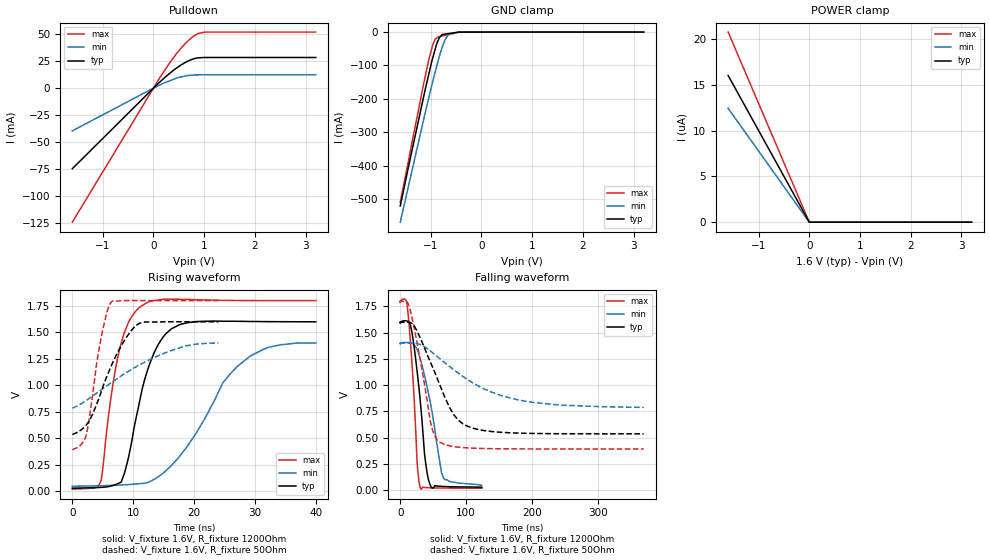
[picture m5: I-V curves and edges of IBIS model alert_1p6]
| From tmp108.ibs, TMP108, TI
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|   alert_1p6 Model
[Model]   alert_1p6
Model_type   Open_drain
Polarity   Non-Inverting
Vmeas = 0.8
Vref = 1.6
Cref = 2pF
Rref = 1200
|   typ   min   max
C_comp   9.597e-13   9.560e-13   1.010e-12
| Where nom  PVT is Nominal Process, 1.6V, 27C
|   Fast PVT is Strong Process,  1.8V, -40C
|   Slow PVT is Weak Process,   1.4V, 125C
[Voltage Range]   1.6   1.4   1.8
|Ambient Temperature   25   125   -40
|Junction Temperature
[Temperature Range]   27   125   -40
[Pullup Reference]   1.6   1.4   1.8
[Pulldown Reference]   0   0   0
[Power Clamp Reference]   1.6   1.4   1.8
[GND Clamp Reference]   0   0   0
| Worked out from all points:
|   slope of the pulldown table from 0 to 0.24 V, typ, clamps not added: 22.7 ohm
|   GND clamp passes 1 mA (typ) near -0.49 V on its own axis
|   falling waveform, V_fixture 1.6V, R_fixture 1200Ohm: 20-80 % time 14.3ns typ, 23.4ns min, 9.76ns max; typ from 1.6 V to 0.029 V
|   rising waveform, V_fixture 1.6V, R_fixture 1200Ohm: 20-80 % time 3.97ns typ, 8.85ns min, 2.96ns max; typ from 0.029 V to 1.6 V
|   falling waveform, V_fixture 1.6V, R_fixture 50Ohm: 20-80 % time 43.9ns typ, 93.8ns min, 23.2ns max; typ from 1.6 V to 0.536 V
|   rising waveform, V_fixture 1.6V, R_fixture 50Ohm: 20-80 % time 4.69ns typ, 10.5ns min, 2.24ns max; typ from 0.536 V to 1.6 V
[Pulldown]
|   Voltage   I(typ)   I(min)   I(max)
-1.6V     -74.82mA   -39.69mA   -124.5mA
138.6mV   6.252mA    3.257mA    10.64mA
316.8mV   13.62mA    6.783mA    23.23mA
466.2mV   19.03mA    9.469mA    32.69mA
651.6mV   24.43mA    11.54mA    42.62mA
777.6mV   26.98mA    12.02mA    47.83mA
880.2mV   28.12mA    12.27mA    50.75mA
1.008V    28.45mA    12.4mA     52.03mA
3.2V      28.45mA    12.4mA     52.03mA
[GND Clamp]
|   Voltage   I(typ)   I(min)   I(max)
-1.6V     -521.1mA   -569.6mA   -510.1mA
-1.132V   -189.2mA   -258mA     -150mA
-1.028V   -120.1mA   -191.2mA   -77.1mA
-955.8mV  -75.45mA   -146.4mA   -36.7mA
-909mV    -50.04mA   -118.5mA   -21.17mA
-880mV    -34.6mA    -101.3mA   -17.58mA
-828.8mV  -16.44mA   -72.82mA   -13.41mA
-771.2mV  -7.347mA   -44.63mA   -11.4mA
-711.2mV  -5.991mA   -21.38mA   -9.299mA
-651mV    -4.63mA    -7.953mA   -7.193mA
-428.4mV  -53.65uA   -105.2uA   -65.19uA
3.2V      0A         0A         0A
[POWER Clamp]
|   Voltage   I(typ)   I(min)   I(max)
-1.6V     16uA       12.42uA    20.73uA
-1.4mV    14.05nA    12.36nA    18.18nA
0V        0A         0A         0A
3.2V      0A         0A         0A
[Ramp]
R_load = 1200
|   typ   min   max
dV/dt_r   0.942888/3.95545e-09   0.811826/8.81647e-09   1.06853/2.94365e-09
dV/dt_f   0.942887/1.4268e-08   0.811797/2.33253e-08   1.06853/9.75656e-09
[Falling Waveform]
V_fixture = 1.6V
V_fixture_min = 1.4V
V_fixture_max = 1.8V
R_fixture = 1200Ohm
|   Time   V(typ)   V(min)   V(max)
0s        1.6V       1.4V       1.8V
8.15ns    1.613V     1.408V     1.815V
11.2ns    1.61V      1.407V     1.725V
19.78ns   1.424V     1.392V     1.017V
25.49ns   1.14V      1.341V     284.8mV
30.24ns   864.6mV    1.256V     28.98mV
38.59ns   259.1mV    1.047V     25.35mV
46.04ns   41.23mV    824.9mV    22.77mV
65.25ns   35.68mV    122.9mV    20.46mV
123.9ns   28.52mV    47mV       19.12mV
[Rising Waveform]
V_fixture = 1.6V
V_fixture_min = 1.4V
V_fixture_max = 1.8V
R_fixture = 1200Ohm
|   Time   V(typ)   V(min)   V(max)
0s        28.52mV    46.95mV    19.12mV
4.74ns    36.13mV    51.72mV    103.1mV
6.2ns     46.66mV    54.29mV    823.6mV
7.56ns    73.25mV    57.38mV    1.289V
9.07ns    279.7mV    62mV       1.574V
10.98ns   826.7mV    70.4mV     1.735V
13.82ns   1.353V     125.1mV    1.803V
17.58ns   1.572V     325.9mV    1.813V
27.14ns   1.605V     1.18V      1.801V
40ns      1.6V       1.4V       1.8V
[Falling Waveform]
V_fixture = 1.6V
V_fixture_min = 1.4V
V_fixture_max = 1.8V
R_fixture = 50Ohm
|   Time   V(typ)   V(min)   V(max)
0s        1.6V       1.4V       1.8V
9.96ns    1.6V       1.4V       1.796V
14.83ns   1.598V     1.4V       1.724V
28.39ns   1.478V     1.391V     1.31V
46.04ns   1.217V     1.325V     646.5mV
58.85ns   1.023V     1.259V     461.1mV
81.98ns   714.5mV    1.145V     414.8mV
114.9ns   583.5mV    1.006V     399.3mV
204.4ns   540.2mV    834.5mV    392.9mV
370ns     536.5mV    788.5mV    392.6mV
[Rising Waveform]
V_fixture = 1.6V
V_fixture_min = 1.4V
V_fixture_max = 1.8V
R_fixture = 50Ohm
|   Time   V(typ)   V(min)   V(max)
0s        536.5mV    786.6mV    392.6mV
2.24ns    621.6mV    855.1mV    524.1mV
2.77ns    663.9mV    875.9mV    681mV
4.56ns    907.2mV    949.3mV    1.396V
5.59ns    1.072V     992mV      1.669V
6.45ns    1.19V      1.027V     1.79V
8.99ns    1.462V     1.124V     1.8V
11.08ns   1.587V     1.194V     1.8V
18.5ns    1.6V       1.371V     1.8V
24ns      1.6V       1.4V       1.8V
